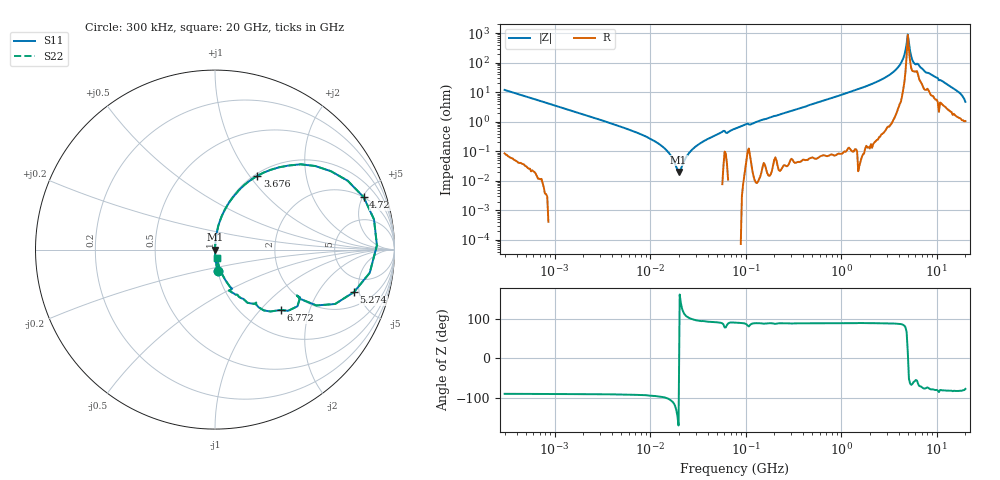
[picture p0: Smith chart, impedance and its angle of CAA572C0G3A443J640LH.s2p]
! S-Parameter Data Generated by TDK Corporation
! Copyright(C) 2022 TDK Corporation.
! All Rights Reserved.
! TDK P/N: CAA572C0G3A443J640LH (Multilayer Ceramic Chip Capacitor)
! Property: C=44nF
! Size(LxWxT): 6x5.6x6.4mm
! Model Type: s2p (Touchstone File Format Version 1.0)
! Frequency: DC=Yes Start=0.3MHz Stop=20000MHz 402points Log-sweep
! Model Generated on Apr. 15, 2022
! Port Assignments:
!  1 ---| |--- 2
! Applicable Conditions:
!  Temperature = 25 degC
!  DC Bias Voltage = 0 V
!  Small Signal Operation
! Terms and conditions regarding TDK Simulation Models
! (1)This simulation model is being provided solely for informational purposes. Please refer to the specifications of the products in terms of detailed characteristics of such products.
! (2)In no event shall TDK Corporation of any of its subsidiaries be liable for any loss or damage arising, directly or indirectly,
!  From any information contained in this simulation model, including, but not limited to loss or damages arising from any inaccuracies, omissions or errors in connection with such information.
! (3)Any and all copyrights on this simulation model are owned by TDK Corporation.
!  Duplication or redistribution of this simulation model without prior written permission from TDK Corporation is prohibited.
! (4)This simulation model is subject to any modification or change without any prior notice.
! (5)Neither TDK Corporation nor any of its subsidiaries shall make any warranty, express or implied,
!  Including but not limited to the correctness, implied warranties of merchantability and fitness for a particular purpose with respect to this simulation models.
! (6)The use of this simulation model shall be deemed to have consented to the terms and conditions hereof.
# Hz S MA R 50
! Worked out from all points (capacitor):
!   401 points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, 300 kHz to 20 GHz, reference 50 ohm
!   read as one part in series: C = 44.4 nF near 317.1 kHz
!   lowest |Z| = 19.8 mohm at 19.87 MHz (marker M1)
!   series resonance near 20.07 MHz, so ESL is about 1.4 nH
!   S11 on the Smith chart (normalised r, x): 300 kHz: 1.00, -0.24; 3.676 GHz: 1.03, +1.09; 4.72 GHz: 1.99, +5.09; 5.274 GHz: 3.21, -4.42; 6.772 GHz: 1.46, -1.30; 20 GHz: 1.02, -0.09
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300000  0.1183 -82.8  0.9921 6.8  0.9921 6.8  0.1183 -82.8
1928084  0.01837 -89.4  1 1.1  1 1.1  0.01837 -89.4
6916326  0.004579 -91.9  1 0.3  1 0.3  0.004579 -91.9
1.239169e7  0.00178 -96.2  1 0.1  1 0.1  0.00178 -96.2
1.590994e7  0.0008435 -103.4  1 0.0  1 0.0  0.0008435 -103.4
1.986766e7  0.0001985 -169.7  1 0.0  1 0.0  0.0001985 -169.7
2.550849e7  0.0008637 102.8  1 -0.0  1 -0.0  0.0008637 102.8
3.098155e7  0.001567 96.3  1 -0.1  1 -0.1  0.001567 96.3
7.964076e7  0.006051 90.3  1 -0.3  1 -0.3  0.006051 90.3
4.978292e8  0.03929 86.8  0.9986 -2.3  0.9986 -2.3  0.03929 86.8
1.643049e9  0.1384 81.8  0.9898 -8.0  0.9898 -8.0  0.1384 81.8
3.199522e9  0.3547 68.2  0.9286 -20.8  0.9286 -20.8  0.3547 68.2
3.676071e9  0.4747 60.1  0.8672 -28.3  0.8672 -28.3  0.4747 60.1
4.342527e9  0.7277 39.8  0.641 -46.6  0.641 -46.6  0.7277 39.8
4.719781e9  0.8783 19.4  0.3391 -59.6  0.3391 -59.6  0.8783 19.4
4.98932e9  0.9025 1.5  0.1007 -13.7  0.1007 -13.7  0.9025 1.5
5.274253e9  0.8096 -17.0  0.3274 46.4  0.3274 46.4  0.8096 -17.0
5.73245e9  0.5829 -29.6  0.5709 30.3  0.5709 30.3  0.5829 -29.6
6.771718e9  0.4968 -42.6  0.718 27.9  0.718 27.9  0.4968 -42.6
9.989315e9  0.2809 -63.6  0.9103 16.0  0.9103 16.0  0.2809 -63.6
1.55773e10  0.1197 -75.4  0.9768 6.8  0.9768 6.8  0.1197 -75.4
2e10  0.04666 -74.5  0.9886 2.6  0.9886 2.6  0.04666 -74.5
